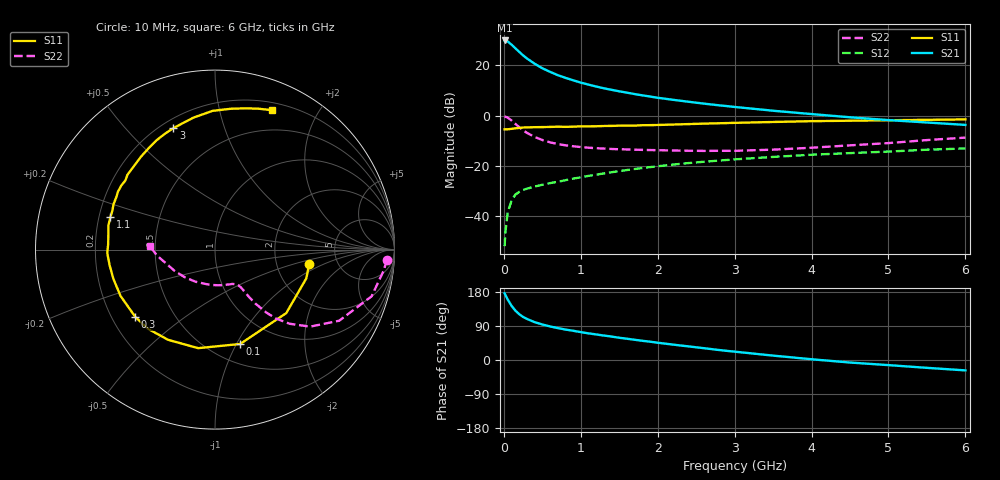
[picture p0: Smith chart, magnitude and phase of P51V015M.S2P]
! SIEMENS Small Signal Semiconductors
! BFP183
! Si NPN RF Bipolar Junction Transistor in SOT143
! VCE = 1 V  IC = 15 mA
! Common Emitter S-Parameters:  March  1996
# GHz  S  MA  R  50
!  f  S11  S21  S12  S22
! GHz  MAG  ANG  MAG  ANG  MAG  ANG  MAG  ANG
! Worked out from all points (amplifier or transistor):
!   36 points, 10 MHz to 6 GHz, reference 50 ohm
!   highest |S21| = 29.9 dB at 10 MHz (marker M1)
!   |S21| within 3 dB of that: start of sweep to 146 MHz
!   unconditionally stable (mu >= 1): 757.8 MHz to end of sweep
!   at 250 MHz: K = 0.46, MSG = 26.8 dB, |S12| = -29.6 dB
!   at 1.4 GHz: K = 1.20, MAG = 13.7 dB, |S12| = -22.6 dB
!   at 6 GHz: K = 1.02, MAG = 3.8 dB, |S12| = -13.1 dB
!   S11 on the Smith chart (normalised r, x): 10 MHz: 3.10, -0.68; 100 MHz: 0.69, -1.03; 300 MHz: 0.30, -0.34; 1.1 GHz: 0.25, +0.14; 3 GHz: 0.25, +0.69; 6 GHz: 0.28, +1.45
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0.01  0.5313 -8.5  31.36 175.9  0.0025 82.4  0.9594 -3.3
0.02  0.5333 -17.5  31.33 172.0  0.0047 84.5  0.9481 -6.9
0.05  0.5318 -41.7  29.94 159.7  0.0118 76.0  0.9106 -16.6
0.1  0.5441 -75.1  25.88 143.1  0.0202 60.9  0.7974 -29.8
0.15  0.5571 -99.7  21.91 130.3  0.0267 53.4  0.682 -39.0
0.2  0.5665 -117.5  18.57 120.9  0.0301 48.2  0.5864 -44.8
0.25  0.578 -130.2  15.82 113.7  0.033 45.5  0.511 -48.6
0.3  0.5812 -139.9  13.75 108.4  0.0349 44.3  0.4524 -50.8
0.4  0.5863 -153.9  10.79 99.9  0.0385 42.9  0.3752 -53.2
0.5  0.5892 -164.0  8.764 93.7  0.0418 42.4  0.3258 -54.3
0.6  0.5938 -171.8  7.442 88.6  0.0451 43.6  0.293 -54.8
0.7  0.6005 -178.1  6.382 84.3  0.0479 44.9  0.271 -55.2
0.8  0.596 176.9  5.65 80.4  0.0515 45.8  0.2555 -55.6
1  0.6094 167.2  4.534 73.6  0.0588 47.3  0.2358 -57.1
1.1  0.61 162.8  4.136 70.3  0.0629 47.6  0.229 -58.2
1.5  0.6297 149.1  3.042 58.7  0.0781 47.8  0.2132 -64.0
2.2  0.6624 128.3  2.061 40.6  0.1054 44.5  0.2011 -80.2
3  0.7156 108.9  1.486 22.0  0.1339 38.4  0.1984 -104.8
3.5  0.7449 99.3  1.248 11.6  0.15 34.0  0.2095 -121.5
4.5  0.7899 83.5  0.924 -6.7  0.1786 25.2  0.255 -152.5
5.5  0.8222 72.7  0.728 -20.7  0.2089 17.4  0.3249 -174.1
6  0.839 67.7  0.651 -27.4  0.2213 12.7  0.3637 176.9
